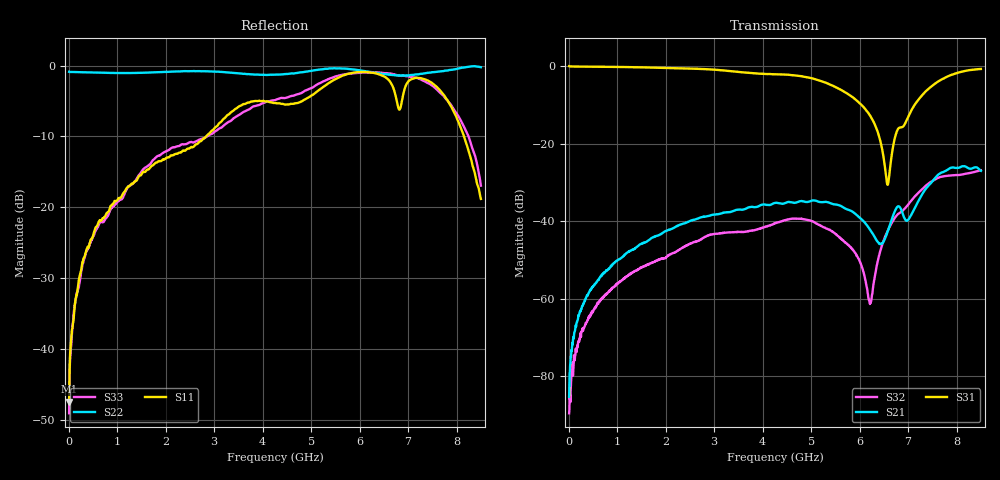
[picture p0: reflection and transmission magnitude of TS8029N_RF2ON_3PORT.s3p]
!Created with skrf (http://scikit-rf.org).
# GHz S RI R 50.0
!freq ReS11 ImS11 ReS12 ImS12 ReS13 ImS13
! ReS21 ImS21 ReS22 ImS22 ReS23 ImS23
! ReS31 ImS31 ReS32 ImS32 ReS33 ImS33
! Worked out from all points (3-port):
!   1601 points, 10 MHz to 8.5 GHz, reference 50 ohm
!   strongest paths, dB at 10 MHz, 2.132 GHz, 4.255 GHz, 6.378 GHz, 8.5 GHz:
!     S31: -0.1, -0.6, -2.1, -17.2, -0.8
!     S21: -85.3, -41.9, -35.3, -45.4, -27.0
!     S32: -89.5, -48.3, -40.6, -50.1, -26.9
!   lowest |S11| = -47.4 dB at 10 MHz (marker M1), VSWR 1.01, Z = 50.2 + j0.392 ohm
!   |S11| at or under -10 dB: start of sweep to 2.834 GHz; 8.151 GHz to end of sweep
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0.01  0.00168 0.00391  -6.34e-06 5.4e-05  0.9931 -0.00926
      3.21e-06 5.44e-05  -0.9044 0.00333  2.99e-05 2.67e-05
      0.993 -0.00928  2.46e-05 2.28e-05  0.00291 0.00197
0.3018438  0.00742 -0.0425  6.91e-05 0.000844  0.9736 -0.1113
           6.67e-05 0.000863  -0.8948 0.073  -5.92e-05 -0.000421
           0.9736 -0.1111  -8.63e-05 -0.00041  0.00338 -0.0405
0.9545125  -0.0267 -0.1078  -0.000298 0.00294  0.9112 -0.3358
           -0.000305 0.00297  -0.8549 0.239  -0.00126 -0.000731
           0.911 -0.3355  -0.00126 -0.000735  -0.0235 -0.1018
4.255  -0.5449 0.0226  0.00844 0.015  -0.0674 -0.7803
       0.00839 0.015  -0.342 0.7933  -0.000417 0.00939
       -0.0687 -0.7787  -0.000398 0.00936  -0.5706 -0.0157
5.491356  -0.5877 0.5437  0.0135 0.0094  -0.3585 -0.4032
          0.0135 0.00943  -0.0469 0.9564  0.00527 0.00453
          -0.3589 -0.4032  0.00524 0.00454  -0.5618 0.6207
6.213006  -0.2342 0.8638  0.00641 0.00445  -0.2073 -0.1004
          0.00642 0.00442  -0.0149 0.9041  -0.000191 0.00084
          -0.2073 -0.1007  -0.000218 0.00083  -0.4281 0.7854
6.573831  0.0831 0.8035  -0.00178 0.00701  -0.00522 -0.029
          -0.00178 0.007  0.0783 0.8627  -0.00714 0.00198
          -0.00523 -0.029  -0.00714 0.00199  -0.0511 0.8826
6.770162  0.1577 0.5294  -0.00161 0.0151  0.1069 -0.098
          -0.00163 0.0151  0.1674 0.8365  -0.0104 0.00605
          0.1071 -0.0978  -0.0104 0.00605  0.2187 0.8267
7.348544  0.458 0.6548  -0.00862 0.0238  0.2967 -0.3521
          -0.00866 0.0239  0.4049 0.7864  -0.0128 0.025
          0.2979 -0.3523  -0.0128 0.025  0.6019 0.4833
8.5  0.0687 0.0917  0.0235 0.0378  -0.2514 -0.8782
     0.0236 0.0378  0.49 0.8431  0.0199 0.0406
     -0.252 -0.8781  0.0199 0.0406  0.1403 0.0235
